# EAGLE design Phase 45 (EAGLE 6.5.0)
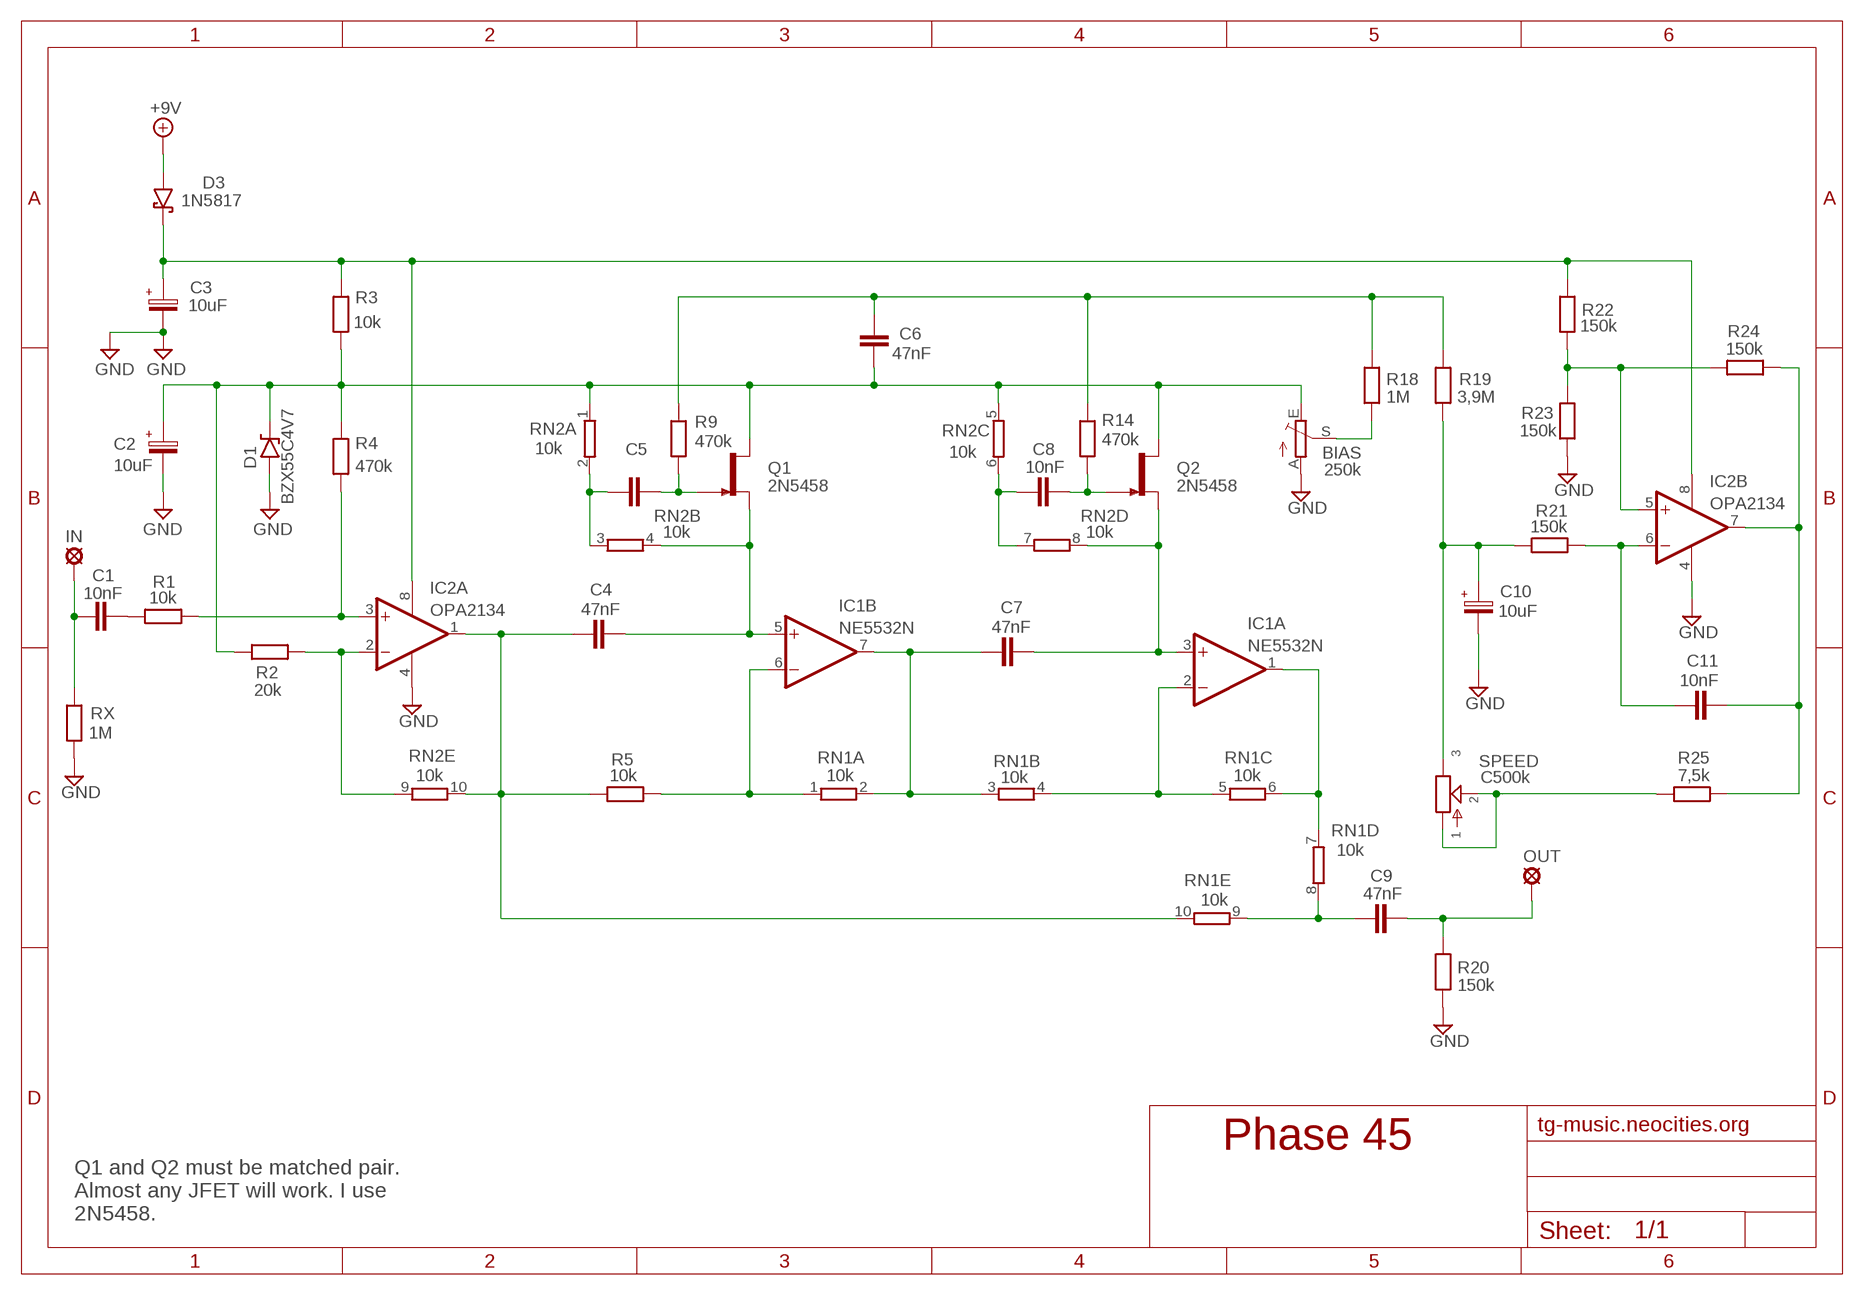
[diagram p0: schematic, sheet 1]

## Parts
+9V  +9V  +9V(T)1  [ROUND]
BIAS  250k  TRIM_EU-PT10  [PT-10]
C1  10nF  1NF-6,8NF  [3,5MM]
C2  10uF  063-EU  [063_025]
C3  10uF  063-EU  [063_025]
C4  47nF  10NF-47NF"  [4,5MM]
C5  10nF  1NF-6,8NF  [3,5MM]
C6  47nF  10NF-47NF"  [4,5MM]
C7  47nF  10NF-47NF"  [4,5MM]
C8  10nF  1NF-6,8NF  [3,5MM]
C9  47nF  10NF-47NF"  [4,5MM]
C10  10uF  063-EU  [063_025]
C11  10nF  1NF-6,8NF  [3,5MM]
D1  BZX55C4V7  1N9ZENER  [DO35-3]
D3  1N5817  [DO41-3]
GND  GND  GND(T)1  [ROUND]
GND11  GND  GND(T)1  [ROUND]
IC1  NE5532N  TL072P  [DIL08]
IC2  OPA2134  TL072P  [DIL08]
IN  MCS10B  [MCS10B]
OUT  MCS10B  [MCS10B]
Q1  2N5458  2N5457  [TO92-]
Q2  2N5458  2N5457  [TO92-]
R1  10k  6MM-EU3  [R0207/3]
R2  20k  6MM-EU3  [R0207/3]
R3  10k  6MM-EU3  [R0207/3]
R4  470k  6MM-EU3  [R0207/3]
R5  10k  6MM-EU3  [R0207/3]
R9  470k  6MM-EU3  [R0207/3]
R14  470k  6MM-EU3  [R0207/3]
R18  1M  6MM-EU3  [R0207/3]
R19  3,9M  6MM-EU3  [R0207/3]
R20  150k  6MM-EU3  [R0207/3]
R21  150k  6MM-EU3  [R0207/3]
R22  150k  6MM-EU3  [R0207/3]
R23  150k  6MM-EU3  [R0207/3]
R24  150k  6MM-EU3  [R0207/3]
R25  7,5k  6MM-EU3  [R0207/3]
RN1  10k  E5R  [SIL10]
RN2  10k  E5R  [SIL10]
RX  1M  6MM-EU3  [R0207/3]
SPEED  C500k  POT-EU16MM  [16MM]

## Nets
+9V: +9V.1(+9V) D3.A
GND: BIAS.A C2.- C3.- C10.- D1.A GND11.1(GND) GND.1(GND) IC1.4(P:V-) IC2.4(P:V-) R20.1 R23.1 RX.1
N$1: IC2.3(A:+IN) R1.2 R4.1
N$2: C1.2 R1.1
N$3: C1.1 IN.MP RX.2
N$4: IC2.2(A:-IN) R2.2 RN2.9
N$5: C4.1 IC2.1(A:OUT) R5.1 RN1.10 RN2.10
N$6: BIAS.E C2.+ C6.1 D1.C Q1.3(D) Q2.3(D) R2.1 R3.1 R4.2 RN2.1 RN2.5
N$7: IC1.6(B:-IN) R5.2 RN1.1
N$8: C5.1 RN2.2 RN2.3
N$9: C4.2 IC1.5(B:+IN) Q1.2(S) RN2.4
N$10: C5.2 Q1.1(G) R9.1
N$11: C7.1 IC1.7(B:OUT) RN1.2 RN1.3
N$12: C8.2 Q2.1(G) R14.1
N$13: C8.1 RN2.6 RN2.7
N$14: C7.2 IC1.3(A:+IN) Q2.2(S) RN2.8
N$15: IC2.5(B:+IN) R22.1 R23.2 R24.1
N$16: IC1.2(A:-IN) RN1.4 RN1.5
N$17: IC1.1(A:OUT) RN1.6 RN1.7
N$18: C9.1 RN1.8 RN1.9
N$19: C9.2 OUT.MP R20.2
N$20: C6.2 R9.2 R14.2 R18.2 R19.2
N$21: BIAS.S R18.1
N$22: C11.2 IC2.7(B:OUT) R24.2 R25.2
N$23: C11.1 IC2.6(B:-IN) R21.2
N$24: C10.+ R19.1 R21.1 SPEED.3
N$25: R25.1 SPEED.1 SPEED.2
N$32: C3.+ D3.C IC1.8(P:V+) IC2.8(P:V+) R3.2 R22.2

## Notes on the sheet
- tg-music.neocities.org
- Q1 and Q2 must be matched pair.
  Almost any JFET will work. I use
  2N5458.

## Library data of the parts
+9V = gm-supply:+9V(T): +9V Voltage Supply
BIAS = pot:TRIM_EU-: POTENTIOMETER
C1 C5 C8 C11 = Mylar Kondensaattorit:1NF-6,8NF: 1nF-6,8nF
C2 C3 C10 = Elektrolyytit:063-EU
C4 C6 C7 C9 = Mylar Kondensaattorit:10NF-47NF: 10nF-47nF
D1 = Diodit:1N9*ZENER: 1N9???B Zener Diode
D3 = Diodit:1N5817
GND GND11 = gm-supply:GND(T): Ground
IC1 IC2 = Operaatiovahvistimet:TL072: OP AMP
IN OUT = Padit:MCS10B: SOLDER PAD
Q1 Q2 = Transistorit:2N5457: N-CHANNEL JFET
R1-R5 R9 R14 R18-R25 RX = Vastukset:6MM-EU: 6mm Resistors (European schematic symbol)
RN1 RN2 = resistor-sil:E5R: SIL RESISTOR; OC_FARNELL: unknown; OC_NEWARK: unknown
SPEED = gm-pots:POT-EU

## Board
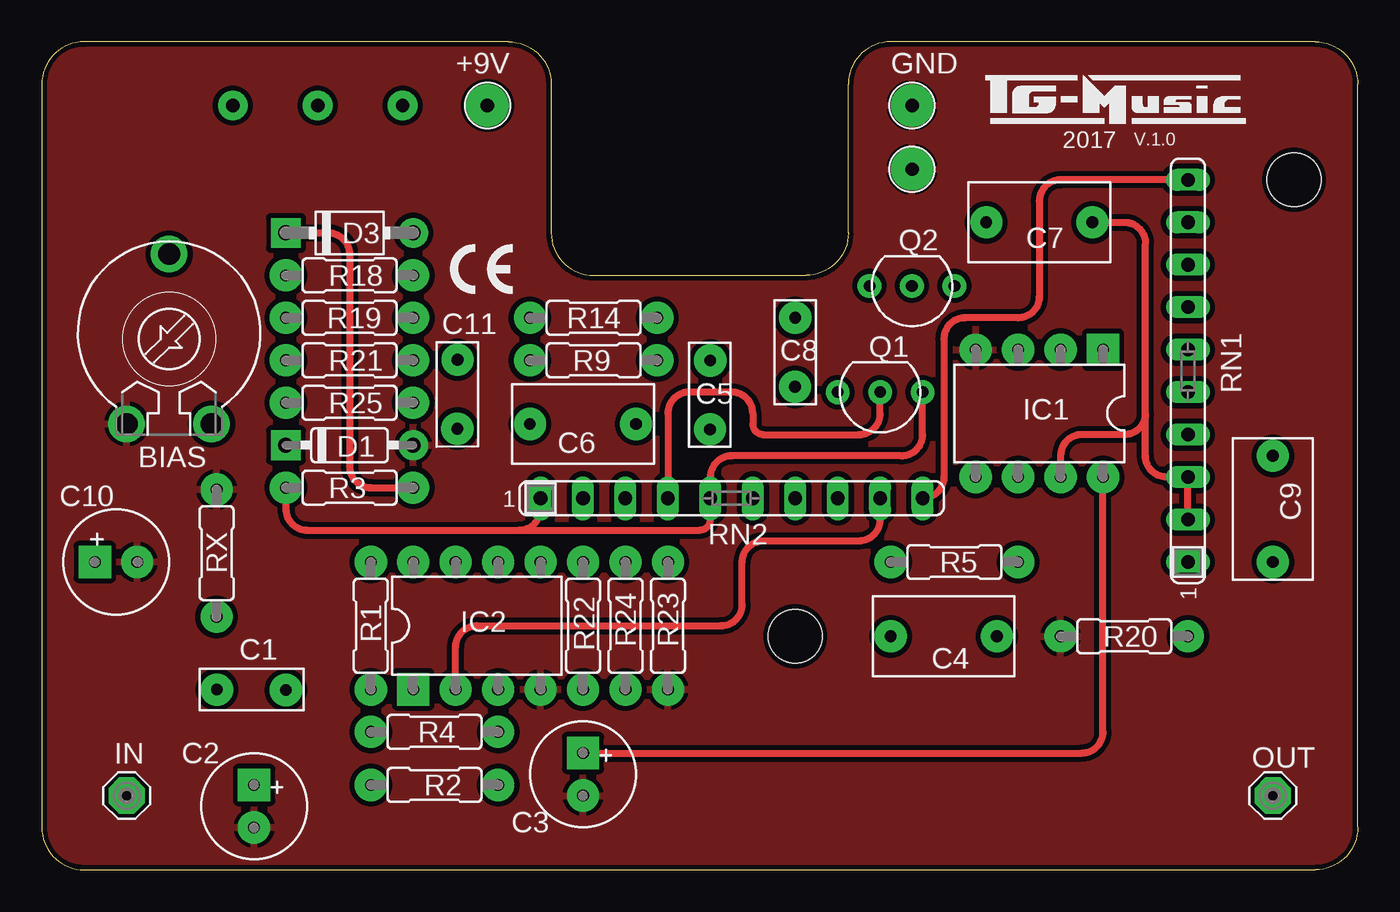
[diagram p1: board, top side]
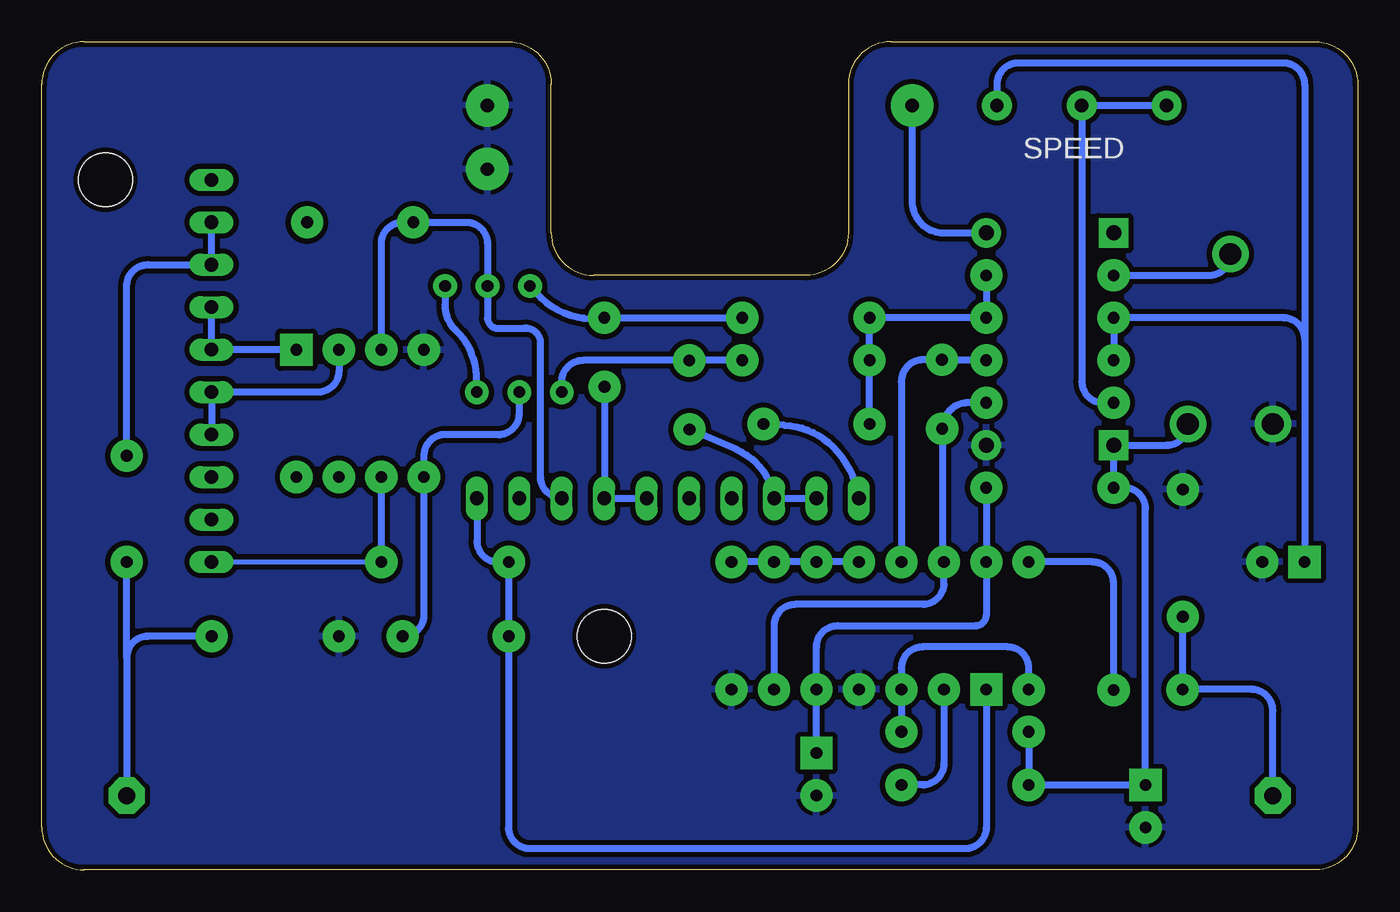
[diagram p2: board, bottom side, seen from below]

Size 78.74 x 49.53 mm. Coordinates in mm from the lower left corner, seen from the top.
Outline: 78.74,2.54 78.74,46.99 arc90 76.2,49.53 50.8,49.53 arc90 48.26,46.99 48.26,38.1 arc-90 45.72,35.56 33.02,35.56 arc-90 30.48,38.1 30.48,46.99 arc90 27.94,49.53 2.54,49.53 arc90 0,46.99 0,2.54 arc90 2.54,0 76.2,0 arc90 78.74,2.54
Copper layers (1*16): Top 0.035mm / dielectric 1.5mm / Bottom 0.035mm
Design rules "ITEADstudio": minimum track width 10mil, minimum drill 12mil, track to track 12mil, track to pad 12mil, pad to pad 12mil, via to via 12mil, smd to smd 0mil, copper to edge 12mil, drill to drill 12mil, minimum pad ring 10mil, minimum via ring 6mil, stop-mask expansion 4mil, vias tented up to drill 100mil, thermal gap 10mil
Holes 3.2 mm at 74.93,41.27 45.09,13.97

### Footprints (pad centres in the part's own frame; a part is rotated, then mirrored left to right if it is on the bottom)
ROUND = drill 0.8 pad 2.54: 1 0,0
PT-10 = drill 1.3 pad 2.184: A -2.54,-5.08; E 2.54,-5.08; S 0,5.08
3,5MM = drill 0.7 pad 1.93: 1 -1.905,0; 2 2.221,-0.016
063_025 = drill 0.7 pad 1.93 square: + -1.27,0 | drill 0.7 pad 1.93: - 1.27,0
4,5MM = drill 0.7 pad 1.93: 1 -3.175,0; 2 3.175,0
DO35-3 = drill 0.9 pad 1.778: A 3.81,0 | drill 0.9 pad 1.778 square: C -3.81,0
DO41-3 = drill 0.9 pad 1.778: A 3.81,0 | drill 0.9 pad 1.778 square: C -3.81,0
DIL08 = drill 0.7 pad 1.93 square: 1 -3.81,-3.81 | drill 0.7 pad 1.93: 2 -1.27,-3.81; 3 1.27,-3.81; 4 3.81,-3.81; 5 3.81,3.81; 6 1.27,3.81; 7 -1.27,3.81; 8 -3.81,3.81
MCS10B = drill 1.016 pad 2.159 octagon: MP 0,0
TO92- = drill 0.7 pad 1.422: 1 2.54,0; 2 0,0; 3 -2.54,0
R0207/3 = drill 0.7 pad 1.93: 1 -3.81,0; 2 3.81,0
SIL10 = drill 0.813 long: 1 -11.43,0; 2 -8.89,0; 3 -6.35,0; 4 -3.81,0; 5 -1.27,0; 6 1.27,0; 7 3.81,0; 8 6.35,0; 9 8.89,0; 10 11.43,0
16MM = drill 0.8 pad 1.778: 1 5.08,0; 2 0,0; 3 -5.08,0

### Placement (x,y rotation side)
+9V  26.67,45.72 0 top
BIAS  7.62,31.75 0 top
C1  12.38,10.78 0 top
C2  12.7,3.81 270 top
C3  32.38,5.71 270 top
C4  53.98,13.97 0 top
C5  39.98,28.25 90 top
C6  32.38,26.67 180 top
C7  59.69,38.73 180 top
C8  45.07,30.8 90 top
C9  73.66,21.59 270 top
C10  4.45,18.41 0 top
C11  24.88,28.61 270 top
D1  18.41,25.4 0 top
D3  18.41,38.1 0 top
GND  52.07,45.72 0 top
GND11  52.07,41.91 0 top
IC1  59.69,27.3 180 top
IC2  26.04,14.61 0 top
IN  5.08,4.45 0 top
OUT  73.66,4.45 0 top
Q1  50.16,28.57 180 top
Q2  52.07,34.92 180 top
R1  19.68,14.61 270 top
R2  23.5,5.08 0 top
R3  18.41,22.86 0 top
R4  23.5,8.26 180 top
R5  54.61,18.41 0 top
R9  33.02,30.48 180 top
R14  33.02,33.02 180 top
R18  18.41,35.56 0 top
R19  18.41,33.02 0 top
R20  64.77,13.97 0 top
R21  18.41,30.48 0 top
R22  32.38,14.61 270 top
R23  37.47,14.61 90 top
R24  34.92,14.61 270 top
R25  18.41,27.94 0 top
RN1  68.58,29.84 90 top
RN2  41.27,22.23 0 top
RX  10.46,18.94 270 top
SPEED  16.51,45.72 180 top

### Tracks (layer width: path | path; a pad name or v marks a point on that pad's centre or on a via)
+9V
  Bottom 0.406: +9V.1 26.67,40.01 arc-90 24.77,38.1 D3.A
GND
  pour Bottom: 0,2.54 0,46.99 arc-90 2.54,49.53 27.94,49.53 arc-90 30.48,46.99 30.48,38.1 arc90 33.02,35.56 45.72,35.56 arc90 48.26,38.1 48.26,46.99 arc-90 50.8,49.53 76.2,49.53 arc-90 78.74,46.99 78.74,2.54 arc-90 76.2,0 2.54,0 arc-90
  pour Top: 0,1.91 0,46.99 arc-90 2.54,49.53 27.94,49.53 arc-90 30.48,46.99 30.48,38.1 arc90 33.02,35.56 45.72,35.56 arc90 48.26,38.1 48.26,46.99 arc-90 50.8,49.53 76.2,49.53 arc-90 78.74,46.99 78.74,2.54 arc-90 76.2,0 1.91,0 arc-90
N$1
  Bottom 0.406: R1.2 19.68,12.06 arc-90 20.95,13.34 26.04,13.34 arc-90 27.3,12.06 IC2.3 R4.1
N$2
  Bottom 0.406: C1.2 14.61,17.14 arc-90 15.88,18.41 R1.1
N$3
  Bottom 0.406: IN.MP 5.08,9.53 arc-90 6.35,10.79 10.46,10.79 arc-90 C1.1 10.48,13.84 arc2 RX.2
N$4
  Top 0.406: IC2.2 24.77,13.34 arc-90 26.04,14.61 40.64,14.61 arc90 41.91,15.88 41.91,18.41 arc-90 43.18,19.68 48.9,19.68 arc90 50.16,20.95 RN2.9
  Bottom 0.406: IC2.2 24.77,6.35 arc90 26.04,5.08 R2.2
N$5
  Top 0.406: RN2.10 arc90 53.98,23.5 53.98,31.75 arc-90 55.24,33.02 58.42,33.02 arc90 59.69,34.29 59.69,40.01 arc-90 60.96,41.27 RN1.10
  Bottom 0.406: IC2.1 22.23,2.54 arc90 23.5,1.27 49.53,1.27 arc90 50.8,2.54 C4.1 R5.1 51.44,18.41 arc90 52.7,19.68 RN2.10
N$6
  Top 0.406: R3.1 14.61,21.59 arc90 15.88,20.32 28.57,20.32 | 28.57,20.32 arc90 29.84,21.59 RN2.1 | Q1.3 52.7,26.04 arc-90 51.44,24.77 41.27,24.77 arc90 40.01,23.5 RN2.5 40.01,20.95 arc-90 39.37,20.32 28.57,20.32
  Bottom 0.406: C6.1 34.29,26.59 arc42 31.44,25.34 arc36 RN2.1 | Q2.3 54.62,33.78 arc-47 53.99,32.31 arc48 52.74,29.25 arc-11 Q1.3 | R4.2 R2.1 C2.+ 12.7,21.59 arc-90 13.97,22.86 R3.1 D1.C 11.43,25.4 arc-90 BIAS.E
N$7
  Bottom 0.305: RN1.1 R5.2
  Bottom 0.406: R5.2 IC1.6
N$8
  Bottom 0.406: RN2.2 RN2.3 arc-58 37.18,25.14 C5.1
N$9
  Top 0.406: RN2.4 37.47,27.3 arc-90 38.73,28.57 41.27,28.57 arc-90 42.55,27.3 42.55,26.67 arc90 43.18,26.04 48.9,26.04 arc90 50.16,27.3 Q1.2
  Bottom 0.406: C4.2 arc-90 55.88,15.24 IC1.5 55.88,24.77 arc90 54.61,26.04 51.44,26.04 arc-90 50.16,27.3 Q1.2
N$10
  Bottom 0.406: R9.1 C5.2 arc-90 C5.2 46.36,30.47 arc-90 47.62,29.21 Q1.1
N$11
  Top 0.406: C7.1 64.77,38.73 arc-90 66.04,37.47 66.04,27.3 | 66.04,27.3 arc-90 64.77,26.04 62.23,26.04 arc90 60.96,24.77 IC1.7 | RN1.2 RN1.3 67.31,23.5 arc-90 66.04,24.77 66.04,27.3
N$12
  Bottom 0.406: R14.1 44.45,33.02 arc90 44.45,33.02 C8.2 arc57 49.16,34.5 Q2.1
N$13
  Bottom 0.406: RN2.6 RN2.7 arc-90 45.07,22.24 C8.1
N$14
  Bottom 0.406: IC1.3 58.42,37.47 arc90 57.15,38.73 C7.2 53.34,38.73 arc90 52.07,37.47 Q2.2 52.07,33.02 arc-90 51.44,32.38 49.9,32.38 arc90 48.9,31.64 48.9,23.58 arc-90 RN2.8
N$15
  Bottom 0.406: IC2.5 R22.1 R24.1 R23.2
N$16
  Bottom 0.406: RN1.4 RN1.5 62.23,28.57 arc-90 60.96,29.84 IC1.2
N$17
  Bottom 0.406: RN1.7 RN1.6 IC1.1
N$18
  Bottom 0.406: RN1.9 RN1.8 72.39,36.2 arc-90 73.66,34.92 C9.1
N$19
  Bottom 0.406: 73.66,12.7 OUT.MP | 73.66,12.7 C9.2 | R20.2 72.39,13.97 arc-90 73.66,12.7
N$20
  Bottom 0.406: R18.2 R19.2 R14.2 R9.2 C6.2
N$21
  Bottom 0.406: R18.1 8.89,35.56 arc-90 BIAS.S
N$22
  Bottom 0.406: R25.2 23.31,27.94 arc-90 C11.2 24.86,18.51 arc-90 IC2.7 24.77,17.14 arc90 26.04,15.88 33.66,15.88 arc-90 34.92,14.61 R24.2
N$23
  Bottom 0.406: R21.2 24.84,30.48 arc90 C11.1 26,30.51 arc-90 27.3,29.21 IC2.6
N$24
  Bottom 0.406: R21.1 R19.1 4.45,33.02 arc90 3.17,31.75 | 3.17,31.75 C10.+ | 3.17,31.75 3.17,46.99 arc-90 4.45,48.26 20.32,48.26 arc-90 21.59,46.99 SPEED.3
N$25
  Bottom 0.406: SPEED.1 SPEED.2 16.51,29.21 arc-90 15.24,27.94 R25.1
N$32
  Top 0.406: D3.C 17.14,38.1 arc-90 18.41,36.83 18.41,24.13 arc90 19.68,22.86 R3.2 | C3.+ 62.23,6.99 arc90 63.5,8.26 IC1.8
  Bottom 0.406: R3.2 IC2.8 22.23,15.24 arc90 22.86,14.61 31.11,14.61 arc-90 32.38,13.34 R22.2 C3.+

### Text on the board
tNames: 2017 | V.1.0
